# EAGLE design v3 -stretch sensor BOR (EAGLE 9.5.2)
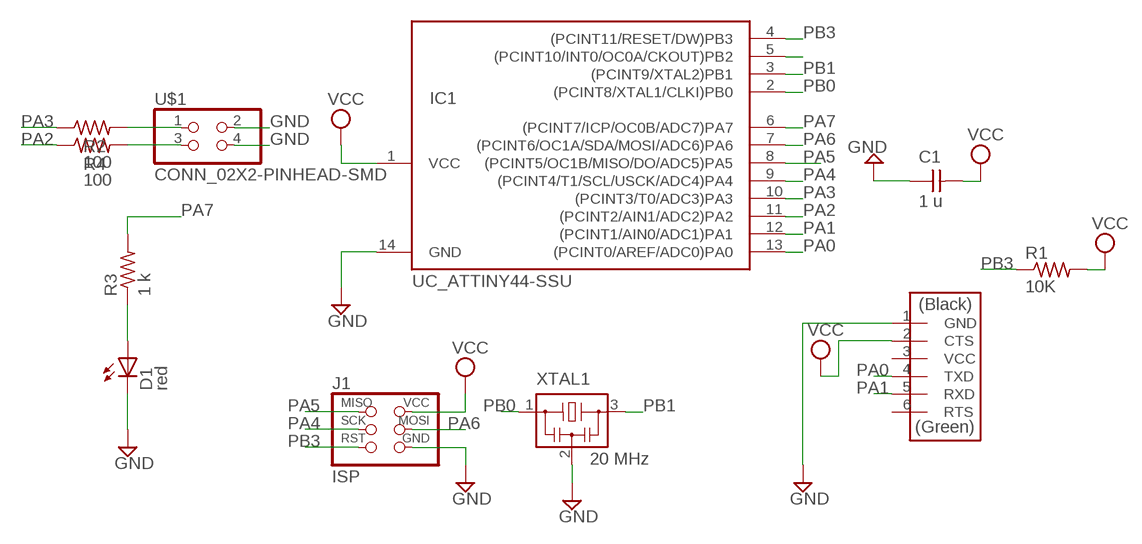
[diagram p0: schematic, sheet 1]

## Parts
C1  1 u  CAP_UNPOLARIZEDFAB  [C1206FAB]
D1  red  LEDFAB1206  [LED1206FAB]
IC1  UC_ATTINY44-SSU  [SOIC14]
J1  ISP  CONN_03X2_AVRISPSMD  [2X03SMD]
J2  FTDI  CONN_06_FTDI-SMD-HEADER  [1X06SMD]
R1  10K  R1206FAB  [R1206FAB]
R2  100  R1206FAB  [R1206FAB]
R3  1 k  R1206FAB  [R1206FAB]
R4  100  R1206FAB  [R1206FAB]
U$1  CONN_02X2-PINHEAD-SMD  [2X02SMD]
XTAL1  20 MHz  XTAL_RESONATOR  [EFOBM]

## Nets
GND: C1.1 D1.2(C) IC1.14(GND) J1.6(GND) J2.1(GND) U$1.2 U$1.4 XTAL1.2
N$1: D1.1(A) R3.1
N$3: R2.2 U$1.1
N$5: R4.2 U$1.3
PA0: IC1.13((PCINT0/AREF/ADC0)PA0) J2.4(TXD)
PA1: IC1.12((PCINT1/AIN0/ADC1)PA1) J2.5(RXD)
PA2: IC1.11((PCINT2/AIN1/ADC2)PA2) R4.1
PA3: IC1.10((PCINT3/T0/ADC3)PA3) R2.1
PA4: IC1.9((PCINT4/T1/SCL/USCK/ADC4)PA4) J1.3(SCK)
PA5: IC1.8((PCINT5/OC1B/MISO/DO/ADC5)PA5) J1.1(MISO)
PA6: IC1.7((PCINT6/OC1A/SDA/MOSI/ADC6)PA6) J1.4(MOSI)
PA7: IC1.6((PCINT7/ICP/OC0B/ADC7)PA7) R3.2
PB0: IC1.2((PCINT8/XTAL1/CLKI)PB0) XTAL1.1
PB1: IC1.3((PCINT9/XTAL2)PB1) XTAL1.3
PB2: IC1.5((PCINT10/INT0/OC0A/CKOUT)PB2)
PB3: IC1.4((PCINT11/RESET/DW)PB3) J1.5(RST) R1.1
VCC: C1.2 IC1.1(VCC) J1.2(VCC) J2.2(CTS) R1.2
Unconnected: J2.3(VCC) J2.6(RTS)

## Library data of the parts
C1 = eagle_fab:CAP_UNPOLARIZED
D1 = eagle_fab:LED: LED
IC1 = eagle_fab:UC_ATTINY44
J1 = eagle_fab:CONN_03X2_AVRISP
J2 = eagle_fab:CONN_06_FTDI-SMD-HEADER
R1-R4 = eagle_fab:R: Resistor (US Symbol)
U$1 = eagle_fab:CONN_02X2-PINHEAD-SMD
XTAL1 = eagle_fab:XTAL_RESONATOR

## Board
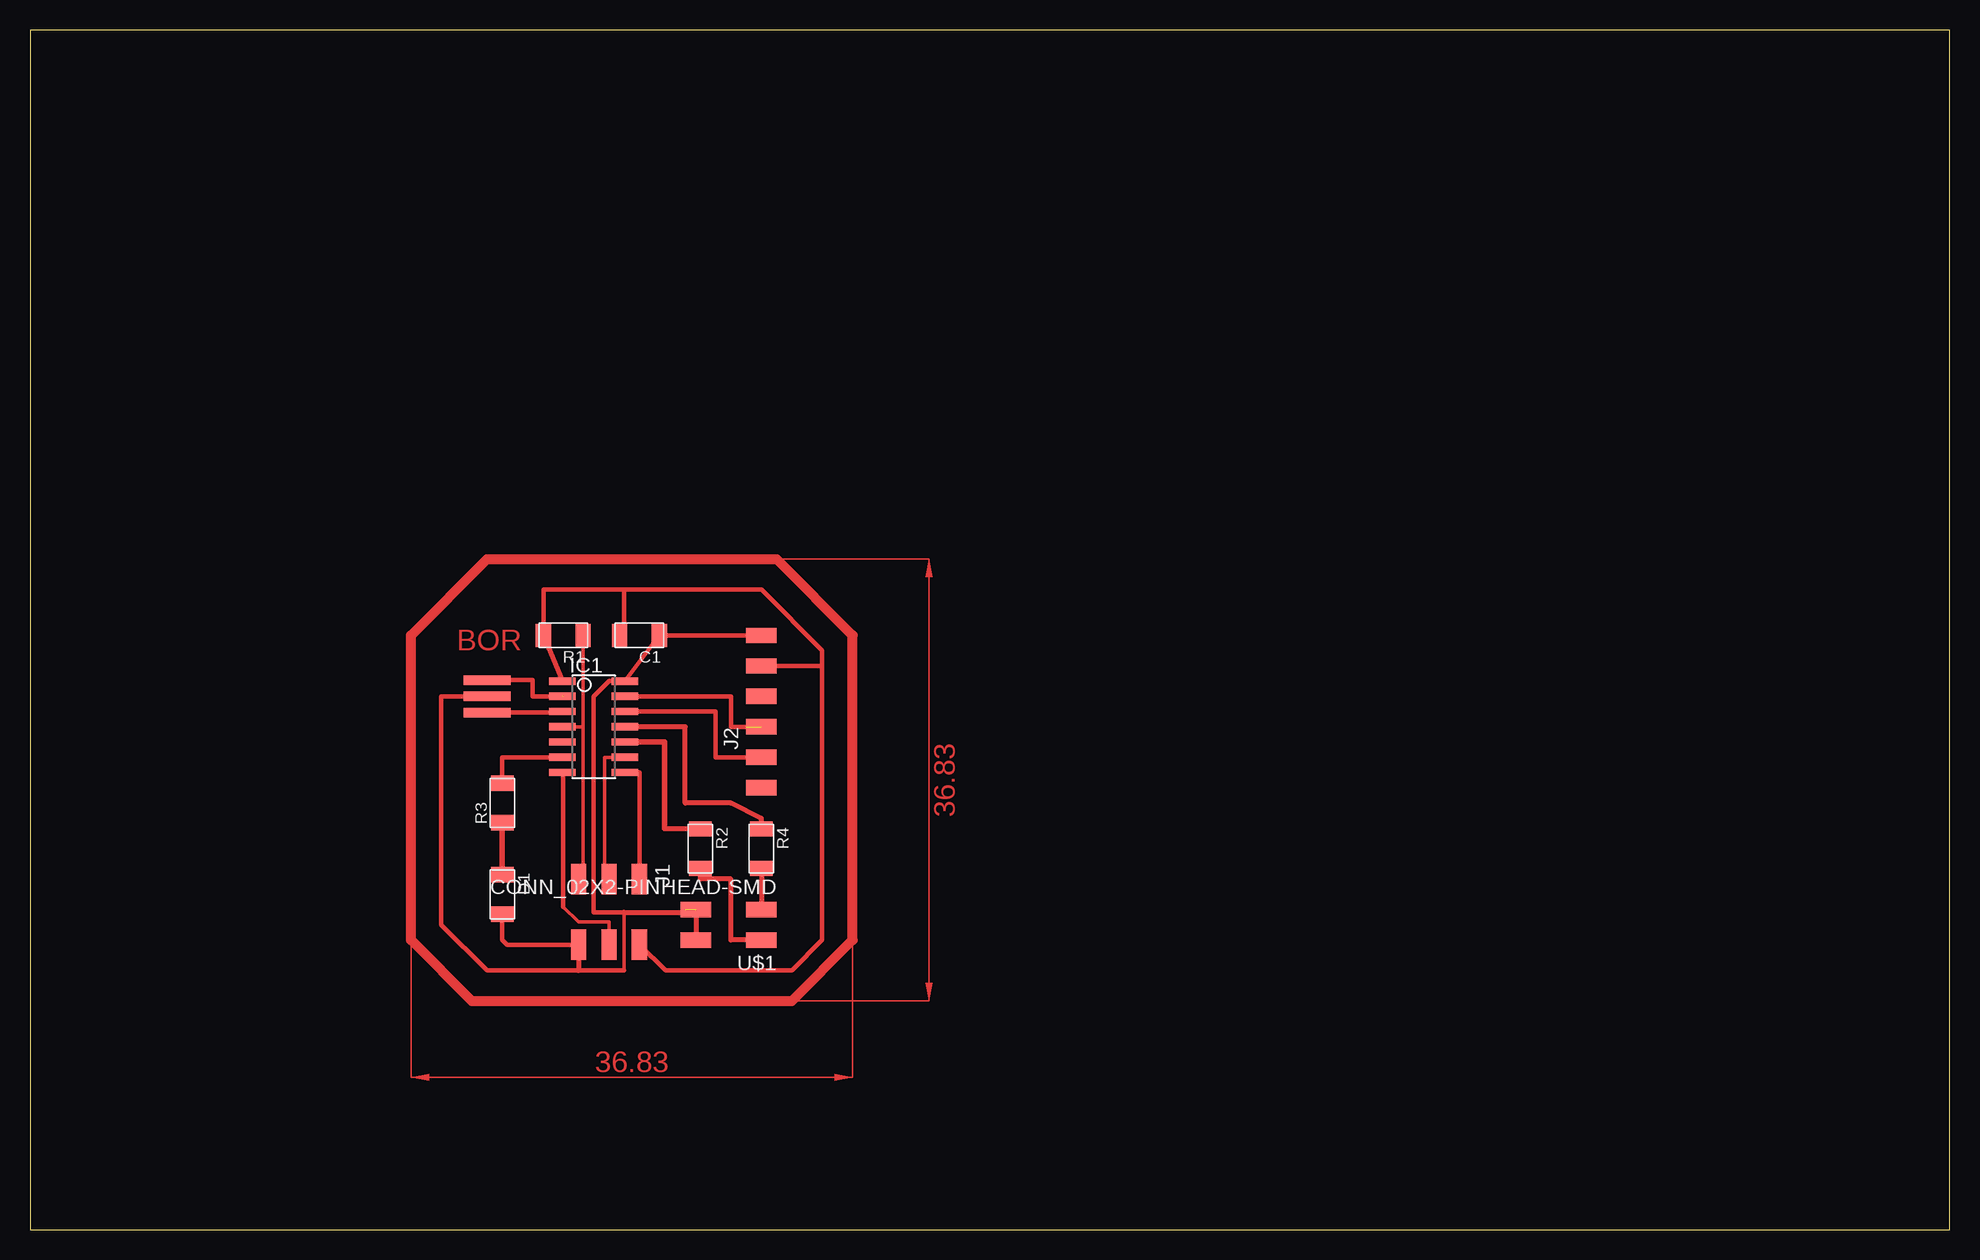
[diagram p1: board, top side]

Size 160 x 100 mm. Coordinates in mm from the lower left corner, seen from the top.
Outline: 0,0 160,0 160,100 0,100 0,0
Copper layers (1*16): Top 0.035mm / dielectric 1.5mm / Bottom 0.035mm
Design rules "default *": minimum track width 10mil, minimum drill 32mil, track to track 18mil, track to pad 18mil, pad to pad 18mil, via to via 18mil, smd to smd 6mil, copper to edge 16mil, drill to drill 16mil, minimum pad ring 10mil, minimum via ring 8mil, stop-mask expansion 4mil, vias tented up to drill 0mil, thermal gap 16mil

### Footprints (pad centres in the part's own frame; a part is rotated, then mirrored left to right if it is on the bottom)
C1206FAB = smd 1.27 x 1.905: 1 -1.651,0; 2 1.651,0
LED1206FAB = smd 1.27 x 1.905: 1 -1.651,0; 2 1.651,0
SOIC14 = smd 0.61 x 2.21: 1 -3.81,-2.603; 2 -2.54,-2.603; 3 -1.27,-2.603; 4 0,-2.603; 5 1.27,-2.603; 6 2.54,-2.603; 7 3.81,-2.603; 8 3.81,2.603; 9 2.54,2.603; 10 1.27,2.603; 11 0,2.603; 12 -1.27,2.603; 13 -2.54,2.603; 14 -3.81,2.603
2X03SMD = smd 2.54 x 1.27: 1 -2.54,2.54; 2 2.92,2.54; 3 -2.54,0; 4 2.92,0; 5 -2.54,-2.54; 6 2.92,-2.54
1X06SMD = smd 2.54 x 1.27: 1 0,6.35; 2 0,3.81; 3 0,1.27; 4 0,-1.27; 5 0,-3.81; 6 0,-6.35
R1206FAB = smd 1.27 x 1.905: 1 -1.651,0; 2 1.651,0
2X02SMD = smd 2.54 x 1.27: 1 -2.54,1.27; 2 2.92,1.27; 3 -2.54,-1.27; 4 2.92,-1.27
EFOBM = smd 0.8 x 3.9: 1 -1.35,0; 2 0,0; 3 1.35,0

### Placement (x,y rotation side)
C1  50.8,49.53 180 top
D1  39.37,27.94 270 top
IC1  46.99,41.91 270 top
J1  48.26,26.67 270 top
J2  60.96,43.18 0 top
R1  44.45,49.53 180 top
R2  55.88,31.75 270 top
R3  39.37,35.56 90 top
R4  60.96,31.75 270 top
U$1  58.42,25.4 180 top
XTAL1  38.1,44.45 270 top

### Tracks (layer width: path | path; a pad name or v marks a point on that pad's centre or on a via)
GND  (1 unrouted)
  Top 0.305: 49.51,21.59 49.51,26.44
  Top 0.356: J2.1 C1.1 IC1.14 48.26,45.72 46.99,44.45 46.99,26.44 49.51,26.44 | 49.51,21.59 45.72,21.59 38.1,21.59 34.29,25.4 34.29,44.45 XTAL1.2 | D1.2 39.37,24.13 39.75,23.75 J1.6
  Top 0.406: J1.6 45.72,21.59 | U$1.4 U$1.2 | 49.51,26.44 54.61,26.44 54.61,26.67
N$1
  Top 0.457: D1.1 R3.1
N$2
  Top 0.813: 38.1,55.88 62.23,55.88 68.58,49.53 68.58,24.13 63.5,19.05 36.83,19.05 31.75,24.13 31.75,49.53 38.1,55.88
N$3
  Top 0.406: U$1.1 58.42,24.13 58.42,29.21 55.88,29.21 R2.2
N$5
  Top 0.406: R4.2 U$1.3
PA0  (1 unrouted)
  Top 0.356: IC1.13 58.42,44.45 58.42,41.91 59.69,41.91
PA1
  Top 0.356: IC1.12 57.15,43.18 57.15,39.37 J2.5
PA2
  Top 0.406: IC1.11 54.61,41.91 54.61,35.56 58.42,35.56 60.96,34.29 R4.1
PA3
  Top 0.406: R2.1 52.88,33.4 52.88,33.78
  Top 0.457: IC1.10 52.88,40.64 52.88,33.78
PA4
  Top 0.254: 47.95,29.21 J1.3
  Top 0.305: IC1.9 47.88,39.37 47.88,29.21
  Top 0.406: 47.88,29.21 J1.3
PA5
  Top 0.356: J1.1 50.8,38.1 IC1.8
PA6
  Top 0.305: J1.4 48.26,25.63 45.72,25.63 44.45,26.9
  Top 0.356: 44.45,26.9 44.45,38.1
  Top 0.406: 44.45,38.1 IC1.7
PA7
  Top 0.356: R3.2 39.37,39.37 IC1.6
PB0  (1 unrouted)
  Top 0.356: XTAL1.1 41.91,45.8 41.91,44.45 44.45,44.45
PB1
  Top 0.356: XTAL1.3 44.39,43.1
  Top 0.406: 44.39,43.1 IC1.3
PB3
  Top 0.305: R1.1 46.1,41.91 | 46.1,41.91 IC1.4 | 46.1,41.91 46.1,29.21
  Top 0.406: 46.1,29.21 J1.5
VCC
  Top 0.356: 49.53,49.53 49.53,53.34 | 49.53,53.34 42.8,53.34 R1.2 IC1.1 | 66.04,46.99 J2.2 | 66.04,46.99 66.04,48.26 60.96,53.34 49.53,53.34 | 66.04,46.99 66.04,24.13 63.5,21.59 52.96,21.59 J1.2
  Top 0.406: 49.53,49.53 C1.2 | J1.2 51.18,24.13
(copper drawn outside any net)
  shapes: Top area x2

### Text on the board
Top: BOR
